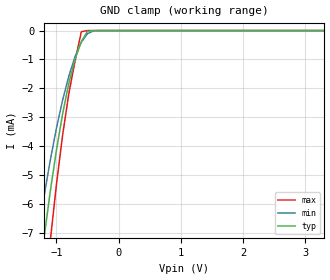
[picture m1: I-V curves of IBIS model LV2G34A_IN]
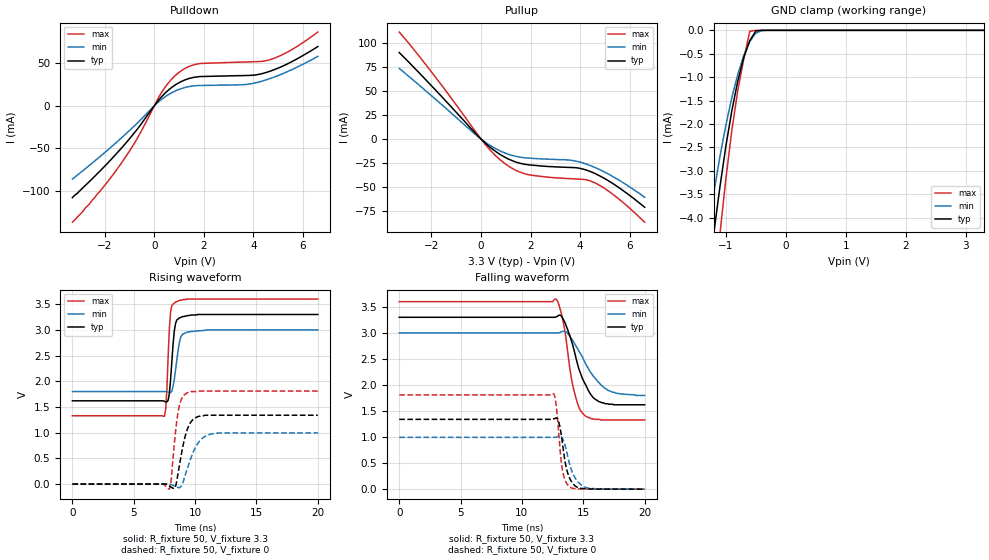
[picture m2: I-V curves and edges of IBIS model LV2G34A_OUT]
|/_/_/_/_/_/_/_/_/_/_/_/_/_/_/_/_/_/_/_/_/_/_/_/_/_/_/_/_/_/_/_/_/_/_/_/_/_/
|   Renesas Electronics Corp.
|   Multi Purpose Semiconductor Digital IC Design Group
|   IBIS Model of HD74LV2G34A
|   3.3V Triple Noninverters,  SSOP-8(8pin) Package
|   History
|   V1.0   April   1, 2003   : First release.
|/_/_/_/_/_/_/_/_/_/_/_/_/_/_/_/_/_/_/_/_/_/_/_/_/_/_/_/_/_/_/_/_/_/_/_/_/_/
[IBIS Ver]   2.1
[Comment Char]  |_char
[File name]   l2g34s3.ibs
[File Rev]   1.1
[Date]   April 1, 2003
[Source]   Data created from SPICE simulations at
|   Renesas Electronics Corp.
[Notes]   RLC value of the Package is determined by assuming typical
|   conditions.
[Disclaimer]   This information is for modeling purposes only, and is not
|   guaranteed.
[Copyright]   Copyright 2003, Renesas Electronics Corp.,
|   All Rights Reserved.
|   Component  HD74LV2G34A
[Component]   HD74LV2G34A
[Manufacturer]  Renesas Electronics Corp.
[Package]
|   typ   min   max
R_pkg   0.099   0.095   0.102
L_pkg   1.740nH   1.680nH   1.790nH
C_pkg   0.140pF   0.140pF   0.150pF
[Pin]   signal_name   model_name   R_pin   L_pin   C_pin
1   1A   LV2G34A_IN   0.102   1.780nH   0.140pF
2   3Y   LV2G34A_OUT   0.097   1.710nH   0.150pF
3   2A   LV2G34A_IN   0.095   1.680nH   0.150pF
4   GND   GND   0.102   1.790nH   0.140pF
5   2Y   LV2G34A_OUT   0.101   1.790nH   0.140pF
6   3A   LV2G34A_IN   0.097   1.710nH   0.150pF
7   1Y   LV2G34A_OUT   0.097   1.710nH   0.150pF
8   VCC   POWER   0.102   1.790nH   0.140pF
| Models and submodels in the file (2): LV2G34A_IN (Input), LV2G34A_OUT (Output)
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|   Model  LV2G34A_IN
[Model]   LV2G34A_IN
Model_type  Input
Vinl = 0.99V
Vinh = 2.31V
| variable   typ   min   max
C_comp   2.35pF   2.25pF   2.45pF
| variable   typ   min   max
[Temperature range]   25   85   -40
| variable   typ   min   max
[Voltage range]   3.3V   3.0V   3.6V
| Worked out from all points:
|   GND clamp passes 1 mA (typ) near -0.70 V on its own axis
[GND Clamp]
|   Voltage   I(typ)   I(min)   I(max)
-3.3V     -64mA      -52mA      -81.2mA
-1.3V     -8.95mA    -7.12mA    -11.9mA
-1.2V     -7.19mA    -5.75mA    -9.48mA
-1.1V     -5.58mA    -4.5mA     -7.3mA
-1V       -4.14mA    -3.38mA    -5.33mA
-900mV    -2.88mA    -2.4mA     -3.61mA
-800mV    -1.82mA    -1.57mA    -2.17mA
-700mV    -976uA     -897uA     -1.05mA
-600mV    -380uA     -405uA     -38.6uA
-500mV    -22.3uA    -104uA     -465nA
-400mV    -445nA     -10.5uA    -2.66nA
3.3V      6.7pA      30.3pA     6.6pA
|   Model  LV2G34A_OUT
[Model]   LV2G34A_OUT
Model_type  Output
Polarity   Inverting
Vmeas = 1.65V
| variable   typ   min   max
C_comp   6.35pF   6.25pF   6.45pF
| variable   typ   min   max
[Temperature range]   25   85   -40
| variable   typ   min   max
[Voltage range]   3.3V   3.0V   3.6V
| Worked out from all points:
|   slope of the pulldown table from 0 to 0.495 V, typ, clamps not added: 29.9 ohm
|   slope of the pullup table from 0 to 0.495 V, typ, clamps not added: 44.6 ohm
|   GND clamp passes 1 mA (typ) near -0.78 V on its own axis
|   rising waveform, R_fixture 50, V_fixture 3.3: 20-80 % time 325ps typ, 422ps min, 255ps max; typ from 1.62 V to 3.3 V
|   rising waveform, R_fixture 50, V_fixture 0: 20-80 % time 724ps typ, 1ns min, 497ps max; typ from 0 V to 1.34 V
|   falling waveform, R_fixture 50, V_fixture 3.3: 20-80 % time 1.41ns typ, 1.93ns min, 944ps max; typ from 3.3 V to 1.62 V
|   falling waveform, R_fixture 50, V_fixture 0: 20-80 % time 605ps typ, 814ps min, 442ps max; typ from 1.34 V to 0 V
[Pullup]
|   Voltage   I(typ)   I(min)   I(max)
-3.3V     89.7mA     73.3mA     111mA
-1.7V     47.1mA     38.3mA     59.6mA
-47.7nV   3.32pA     32.8pA     3.6pA
500mV     -11.2mA    -8.69mA    -15mA
1V        -19.4mA    -14.8mA    -26.2mA
1.5V      -24.6mA    -18.5mA    -33.6mA
1.9V      -26.7mA    -19.7mA    -36.9mA
3.6V      -29.5mA    -21.9mA    -41.1mA
4V        -30.5mA    -24mA      -41.7mA
4.5V      -34.7mA    -28.5mA    -44.4mA
5.3V      -45.9mA    -38.7mA    -57mA
6.6V      -70.8mA    -60.4mA    -86.3mA
[Pulldown]
|   Voltage   I(typ)   I(min)   I(max)
-3.3V     -108mA     -86.2mA    -137mA
-2.2V     -77.1mA    -60mA      -101mA
-1.3V     -49mA      -37.1mA    -66.4mA
-700mV    -28.1mA    -20.8mA    -39.2mA
300mV     10.8mA     7.71mA     15.9mA
1V        27.3mA     19.4mA     39.4mA
1.5V      32.9mA     23.2mA     47.5mA
1.9V      34.6mA     24mA       50mA
3.7V      35.8mA     25.2mA     51.7mA
4.6V      40.1mA     31.4mA     53.8mA
5.4V      49.8mA     40.7mA     63.7mA
6.6V      69.9mA     58.3mA     86.9mA
[GND Clamp]
|   Voltage   I(typ)   I(min)   I(max)
-3.3V     -38.9mA    -31.6mA    -49.2mA
-1.3V     -5.4mA     -4.31mA    -7.13mA
-1.2V     -4.33mA    -3.47mA    -5.69mA
-1.1V     -3.36mA    -2.71mA    -4.37mA
-1V       -2.48mA    -2.03mA    -3.18mA
-900mV    -1.72mA    -1.44mA    -2.14mA
-800mV    -1.08mA    -936uA     -1.28mA
-700mV    -575uA     -533uA     -610uA
-600mV    -219uA     -237uA     -20.5uA
-500mV    -12.9uA    -58.6uA    -245nA
-400mV    -248nA     -6.13uA    -1.4nA
3.3V      3.42pA     32.9pA     3.3pA
[Ramp]
| variable   typ   min   max
dV/dt_r   0.805/724.8p   0.597/1.003n   1.087/497.4p
dV/dt_f   1.010/1.412n   0.718/1.898n   1.362/944.2p
R_load = 50ohms
[Rising Waveform]
R_fixture = 50
V_fixture = 3.3
V_fixture_min = 3.0
V_fixture_max = 3.6
C_fixture = 0p
|   Time   V(typ)   V(min)   V(max)
0s        1.62V      1.8V       1.33V
7.5ns     1.61V      1.8V       1.32V
7.6ns     1.6V       1.8V       1.45V
7.7ns     1.6V       1.8V       1.85V
7.9ns     1.76V      1.78V      3.02V
8ns       2.03V      1.78V      3.35V
8.4ns     3.12V      2.21V      3.54V
8.8ns     3.24V      2.84V      3.58V
9.4ns     3.28V      2.96V      3.6V
20ns      3.3V       3V         3.6V
[Rising Waveform]
R_fixture = 50
V_fixture = 0
C_fixture = 0p
|   Time   V(typ)   V(min)   V(max)
0s        321pV      675nV      144pV
7.9ns     -32.8mV    1.81mV     -99mV
8ns       -51.6mV    -3.3mV     -24mV
8.4ns     -50.7mV    -48.1mV    1.01V
8.7ns     336mV      -71.7mV    1.51V
9.1ns     845mV      102mV      1.73V
9.5ns     1.14V      399mV      1.79V
10.3ns    1.32V      820mV      1.81V
11.3ns    1.34V      973mV      1.81V
20ns      1.34V      995mV      1.81V
[Falling Waveform]
R_fixture = 50
V_fixture = 3.3
V_fixture_min = 3.0
V_fixture_max = 3.6
C_fixture = 0p
|   Time   V(typ)   V(min)   V(max)
0s        3.3V       3V         3.6V
12.8ns    3.31V      3V         3.65V
13.2ns    3.33V      3.02V      3.38V
13.5ns    3.2V       3.03V      3.04V
14.1ns    2.8V       2.87V      2.04V
14.8ns    2.21V      2.59V      1.5V
15.6ns    1.82V      2.24V      1.36V
16.2ns    1.69V      2.06V      1.34V
17.4ns    1.63V      1.86V      1.33V
20ns      1.62V      1.8V       1.33V
[Falling Waveform]
R_fixture = 50
V_fixture = 0
C_fixture = 0p
|   Time   V(typ)   V(min)   V(max)
0s        1.34V      994mV      1.81V
12.6ns    1.35V      995mV      1.83V
12.8ns    1.37V      1V         1.59V
13ns      1.29V      1.01V      1.07V
13.3ns    884mV      976mV      363mV
13.5ns    545mV      856mV      185mV
13.8ns    260mV      560mV      61.3mV
14.4ns    51.3mV     191mV      9.64mV
15.2ns    8.04mV     33.9mV     1.31mV
20ns      -86.7uV    -135uV     -33.1uV
